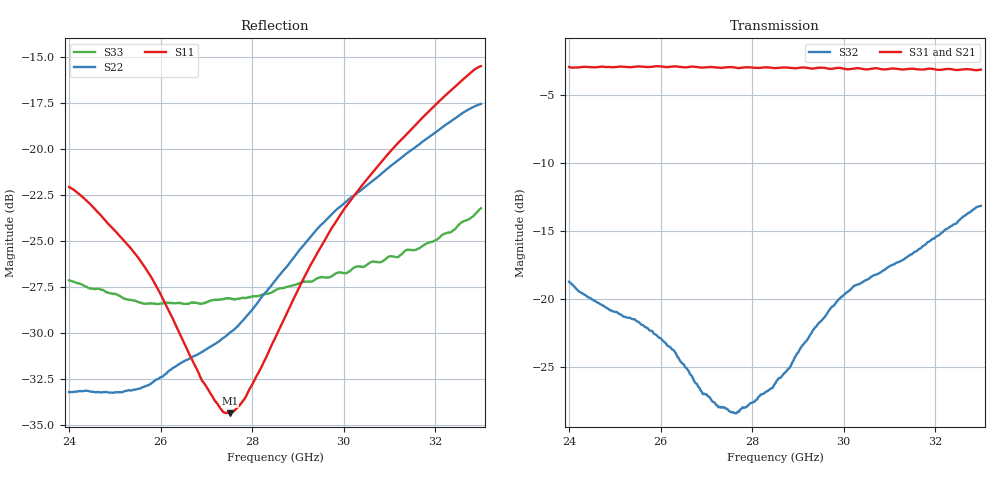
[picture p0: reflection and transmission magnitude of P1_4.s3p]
!The following data was pulled from an Agilent PNA
!This sNp file was generated from the data in the RF Test software
!NOTE:  Smoothing/Math/Corrections applied on any given trace ARE included in the data saved here
# MHz S dB R 50
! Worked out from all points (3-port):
!   1601 points, 24 GHz to 33 GHz, reference 50 ohm
!   strongest paths, dB at 24 GHz, 26.25 GHz, 28.5 GHz, 30.75 GHz, 33 GHz:
!     S31: -3.0, -2.9, -3.1, -3.1, -3.2
!     S21: -3.0, -3.0, -3.0, -3.2, -3.3
!     S32: -18.7, -23.7, -26.2, -18.1, -13.2
!   lowest |S11| = -34.4 dB at 27.52 GHz (marker M1), VSWR 1.04, Z = 50.6 + j1.84 ohm
!   |S11| at or under -10 dB: start of sweep to end of sweep
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24000  -22.07 29.8  -3.11 152.6  -3.07 154.5
       -3.02 152.6  -33.22 155.1  -18.72 102.7
       -2.97 154.2  -18.71 102.4  -27.14 -124.3
25524.38  -25.96 25.2  -3.14 137.4  -3.06 139.4
          -3.06 137.8  -33.04 148.9  -21.69 78.3
          -2.93 139.5  -21.68 78.1  -28.34 -124.4
26289.38  -29.36 28.9  -3.12 130.0  -3.03 131.9
          -3.06 130.0  -31.89 149.2  -23.74 54.3
          -2.92 131.8  -23.76 54.1  -28.38 -124.2
26902.5  -32.59 41.7  -3.09 124.0  -3.01 125.8
         -3.03 123.7  -31.04 147.5  -26.80 34.7
         -3.01 125.4  -26.81 34.5  -28.41 -125.0
27515.62  -34.38 71.8  -3.09 117.3  -3.01 119.2
          -3.11 117.6  -29.98 148.1  -28.23 13.2
          -2.98 119.3  -28.23 13.0  -28.12 -128.6
27847.5  -33.54 91.2  -3.09 113.9  -3.01 115.8
         -3.08 114.1  -29.18 149.6  -27.89 0.3
         -2.99 116.1  -27.92 0.0  -28.11 -130.8
28500  -30.29 115.3  -3.13 107.3  -3.06 109.1
       -3.04 107.6  -27.17 149.0  -26.21 -30.8
       -3.05 109.3  -26.21 -30.9  -27.70 -136.1
29945.62  -23.52 129.0  -3.18 92.0  -3.12 94.0
          -3.17 92.8  -23.11 137.3  -19.81 -83.7
          -3.05 94.2  -19.84 -83.9  -26.72 -158.3
31436.25  -19.05 124.3  -3.19 76.0  -3.13 78.3
          -3.21 76.3  -20.15 122.9  -16.76 -115.2
          -3.10 79.0  -16.77 -115.3  -25.48 167.3
33000  -15.50 115.6  -3.37 59.0  -3.26 61.4
       -3.25 59.4  -17.55 107.4  -13.09 -138.9
       -3.16 62.2  -13.15 -138.9  -23.23 131.1
